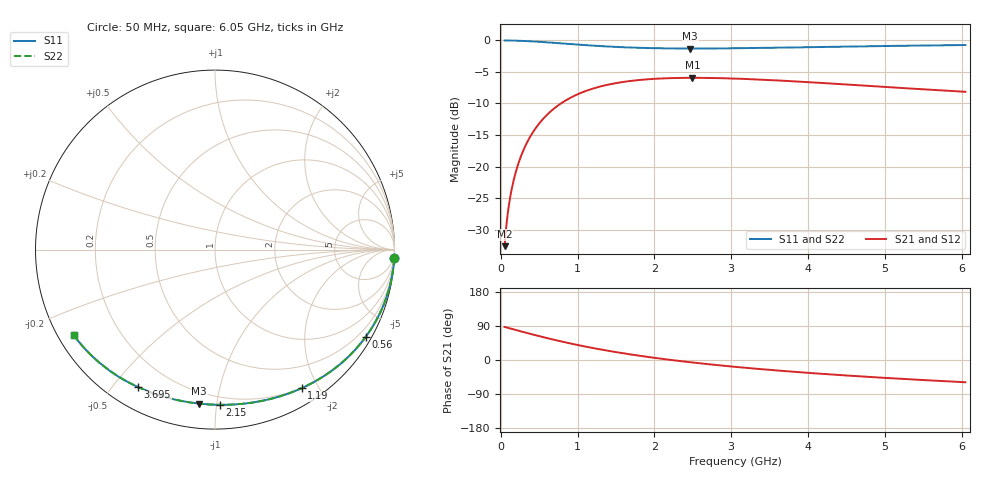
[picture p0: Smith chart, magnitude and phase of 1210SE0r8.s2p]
! AVX Thin Film Operation		Date: August 2001
! Description: Accu-P® Series, Thin Film, SMD, RF Capacitor
! Part Number: 12101J0R8ABT
! 50 MHz  -  6.05 GHz
! Serial Measurements
# mhz S db R 50
!	S11		S21		S12		S22
!	dB	Phase	dB	Phase	dB	Phase	dB	Phase
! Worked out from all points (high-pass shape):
!   401 points, 50 MHz to 6.05 GHz, reference 50 ohm
!   highest |S21| = -5.93 dB at 2.495 GHz (marker M1); lowest = -32.6 dB at 50 MHz (marker M2)
!   |S21| within 3 dB of the highest: 933.6 MHz to end of sweep
!   lowest |S11| = -1.3 dB at 2.465 GHz (marker M3), VSWR 13.56, Z = 6.66 - j44.7 ohm
!   |S11| at or under -10 dB: nowhere
!   |S22| runs from -1.3 to 0.0 dB; largest |S21 - S12| = 0
!   S11 on the Smith chart (normalised r, x): 50 MHz: 0, -41; 560 MHz: 0.22, -3.71; 1.19 GHz: 0.20, -1.79; 2.15 GHz: 0.15, -1.02; 3.695 GHz: 0.09, -0.58; 6.05 GHz: 0.05, -0.28
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50  -0.00 -2.8  -32.64 87.2  -32.64 87.2  -0.00 -2.8
65  -0.00 -3.6  -30.36 86.4  -30.36 86.4  -0.00 -3.6
110  -0.01 -6.1  -25.81 83.9  -25.81 83.9  -0.01 -6.1
140  -0.02 -7.8  -23.73 82.2  -23.73 82.2  -0.02 -7.8
185  -0.03 -10.2  -21.35 79.8  -21.35 79.8  -0.03 -10.2
230  -0.05 -12.7  -19.50 77.3  -19.50 77.3  -0.05 -12.7
290  -0.08 -16.0  -17.55 74.0  -17.55 74.0  -0.08 -16.0
365  -0.12 -20.0  -15.67 70.0  -15.67 70.0  -0.12 -20.0
560  -0.26 -30.1  -12.33 59.9  -12.33 59.9  -0.26 -30.1
785  -0.46 -40.9  -9.98 49.1  -9.98 49.1  -0.46 -40.9
1055  -0.70 -52.6  -8.26 37.4  -8.26 37.4  -0.70 -52.6
1190  -0.81 -58.0  -7.67 32.0  -7.67 32.0  -0.81 -58.0
1610  -1.09 -72.8  -6.55 17.2  -6.55 17.2  -1.09 -72.7
2060  -1.24 -85.9  -6.05 4.1  -6.05 4.1  -1.24 -85.8
2150  -1.26 -88.2  -6.00 1.8  -6.00 1.8  -1.26 -88.2
2465  -1.28 -95.8  -5.93 -5.8  -5.93 -5.8  -1.28 -95.8
2495  -1.28 -96.5  -5.93 -6.5  -5.93 -6.5  -1.28 -96.5
3050  -1.24 -108.0  -6.05 -18.0  -6.05 -18.0  -1.24 -108.0
3695  -1.13 -119.2  -6.40 -29.2  -6.40 -29.2  -1.13 -119.2
4055  -1.06 -124.7  -6.65 -34.7  -6.65 -34.7  -1.06 -124.7
5060  -0.87 -137.8  -7.42 -47.9  -7.42 -47.9  -0.87 -137.8
6050  -0.73 -148.7  -8.15 -58.7  -8.15 -58.7  -0.73 -148.7
